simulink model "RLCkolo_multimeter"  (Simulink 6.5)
settings: Solver=ode45  StartTime=0.0  StopTime=1  RelTol=1e-6
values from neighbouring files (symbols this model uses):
  A = [-R/L -1/L; 1/C 0]    [primer_7_4c.m]
  C = str2num(C)    [patuvacki_bran_1.m]    (also in primer_7_3.m = 0.0001; primer_7_4.m = 0.0001; primer_7_4a.m = 0.0001; primer_7_4c.m = 0.0001)
undefined symbols (not defined in the file or in its folder): B, blocks, Continuous, D, powergui, x0, ZData
libraries: powerlib x8

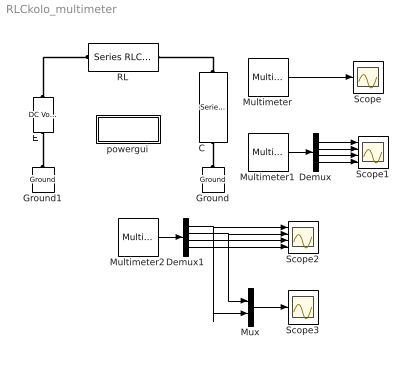
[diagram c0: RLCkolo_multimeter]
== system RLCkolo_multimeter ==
  C : powerlib/Elements/Series RLC Branch  Orientation=down  DialogController=PMDialogs.PMDefaultMaskDlg  PhysicalDomain=powersysdomain  SubClassName=unknown  LeftPortType=p1  RightPortType=p1  LConnTagsString=__new0  RConnTagsString=__new0  BranchType=C  Resistance=1  Inductance=1e-3  SetiL0=off  InitialCurrent=0  Capacitance=100e-6  Setx0=on  InitialVoltage=0  Measurements=Branch voltage and current
  Demux : Demux
  Demux1 : Demux
  E : powerlib/Electrical Sources/DC Voltage Source  Orientation=up  DialogController=PMDialogs.PMDefaultMaskDlg  SystemSampleTime=-1  Amplitude=12  Measurements=None
  Ground : powerlib/Elements/Ground  Orientation=down  DialogController=PMDialogs.PMDefaultMaskDlg  PhysicalDomain=powersysdomain  SubClassName=unknown  LeftPortType=p1  RightPortType=p1  LConnTagsString=a
  Ground1 : powerlib/Elements/Ground  Orientation=down  DialogController=PMDialogs.PMDefaultMaskDlg  PhysicalDomain=powersysdomain  SubClassName=unknown  LeftPortType=p1  RightPortType=p1  LConnTagsString=a
  Multimeter : powerlib/Measurements/Multimeter  SystemSampleTime=-1  PhasorSimulation=off  OutputType=Complex  sel=[1 2 3 4]  L=4  Gain=[1 1 1 1]  yselected={'Ub: C','Ub: RL','Ib: C','Ib: RL'};  PSBOutputType=1  PSBequivalent=0  AxesSetting=[0,0.1,-100,100]  Display=0  SavedBlockNames=-11
  Multimeter1 : powerlib/Measurements/Multimeter  SystemSampleTime=-1  PhasorSimulation=off  OutputType=Complex  sel=[1 2 3 4]  L=4  Gain=[1 1 1 1]  yselected={'Ub: C','Ub: RL','Ib: C','Ib: RL'};  PSBOutputType=1  PSBequivalent=0  AxesSetting=[0,0.1,-100,100]  Display=0  SavedBlockNames=-11
  Multimeter2 : powerlib/Measurements/Multimeter  SystemSampleTime=-1  PhasorSimulation=off  OutputType=Complex  sel=[1 2 3 4]  L=4  Gain=[1 1 1 1]  yselected={'Ub: C','Ub: RL','Ib: C','Ib: RL'};  PSBOutputType=1  PSBequivalent=0  AxesSetting=[0,0.1,-100,100]  Display=0  SavedBlockNames=-11
  Mux : Mux  Inputs=2
  RL : powerlib/Elements/Series RLC Branch  DialogController=PMDialogs.PMDefaultMaskDlg  PhysicalDomain=powersysdomain  SubClassName=unknown  LeftPortType=p1  RightPortType=p1  LConnTagsString=__new0  RConnTagsString=__new0  BranchType=RL  Resistance=3.6  Inductance=0.57  SetiL0=on  InitialCurrent=0  Capacitance=100e-6  Setx0=on  InitialVoltage=0  Measurements=Branch voltage and current
  Scope : Scope
  Scope1 : Scope  NumInputPorts=4
  Scope2 : Scope  NumInputPorts=4
  Scope3 : Scope
  powergui : Subsystem  AncestorBlock=powerlib/powergui  InitFcn=powergui( 'InitFcn_Callback' , gcb , 0 , [ ] );  mask(PSB option menu block){SimulationMode=Continuous, SampleTime=50e-6, echomessages=off, RestoreLinks=warning, x0status=blocks, Frange=[0:2:500], Ylog=off, Xlog=on, ShowGrid=off, save=off, variable=ZData, structure=, ZoomFFT=on, StartTime=0.0, cycles=1, DisplayStyle=1, fundamental=60, FreqAxis=off, MaxFrequency=1000, frequencyindice=0, frequencyindicesteady=1, RmsSteady=1, display=off, Ts=0, frequency=60, methode=off, HookPort=off, Interpol=off}
      mask prompts: SimulationMode "Simulation mode"; SampleTime "Sample time Ts (when simulation mode is Discrete) (s)"; echomessages "Echo  Messages"; RestoreLinks "Restore disabled links"; x0status "Initial electrical states status"; Frange "Impedance tool: Frequency Range"; Ylog "Impedance tool: Log impedance"; Xlog "Impedance tool: log Frequency"; ShowGrid "Impedance tool: grid"; save "Impedance tool: Save Data To Workspace"; variable "Impedance tool: Variable Name"; structure "Structure Name (PSBFFTSCOPE)"; ZoomFFT "ZoomFFT (PSBFFTSCOPE)"; StartTime "Start Time (PSBFFTSCOPE)"; cycles "Cycles (PSBFFTSCOPE)"; DisplayStyle "Display style (PSBFFTSCOPE)"; fundamental "Fundamental (PSBFFTSCOPE)"; FreqAxis "Frequency Axis (PSBFFTSCOPE)"; MaxFrequency "Max Frequency (PSBFFTSCOPE)"; frequencyindice "Load flow frequency (Hz)"; frequencyindicesteady "Frequency indice (STEADYSTATE)"; RmsSteady "RMS display (STEADYSTATE)"; display "Display Results"; Ts "OBSOLETE 1"; frequency "Phasor frequency (Hz)"; methode "Phasor simulation"; HookPort "Hook port"; Interpol "Interpolate"
      mask init:
      | powerlibroot = which('powersysdomain');
      | PSBroot = powerlibroot(1:end-16);
      | %
      | switch SimulationMode
      | 	case 1
      | 		message=sprintf('Continuous');
      | 	case 2
      |         SampleTimeeval=evalin('base',SampleTime,'NaN');
      |         if isnan(SampleTimeeval)
      |             message=sprintf('Warning !!,\nUndefined sample time');
      |         else
      |             message=sprintf('Discrete,\nTs = %.4g s.',SampleTimeeval);
      |         end
      | 	case 3
      | 		message=sprintf('Phasors');
      | end
      | if strcmp(bdroot,'powerlib')
      |   message='powergui';
      | end
      | power_initmask();
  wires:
  Multimeter/1 -> Scope/1
  Multimeter1/1 -> Demux/1
  Demux/1 -> Scope1/1
  Demux/2 -> Scope1/2
  Demux/3 -> Scope1/3
  Demux/4 -> Scope1/4
  Multimeter2/1 -> Demux1/1
  Demux1/1 -> Scope2/1, Mux/2
  Demux1/2 -> Scope2/2, Mux/1
  Demux1/3 -> Scope2/3
  Demux1/4 -> Scope2/4
  Mux/1 -> Scope3/1
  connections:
  C/LConn1 -- RL/RConn1
  E/RConn1 -- RL/LConn1
  Ground/LConn1 -- C/RConn1
  Ground1/LConn1 -- E/LConn1

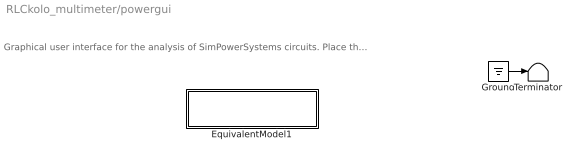
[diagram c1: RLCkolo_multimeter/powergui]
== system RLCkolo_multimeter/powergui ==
  note: Graphical user interface for the analysis of SimPowerSystems circuits. Place the Powergui block in the top-level of your model and double-click on it to open the GUI.
  EquivalentModel1 : Subsystem
  Ground : Ground
  Terminator : Terminator
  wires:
  Ground/1 -> Terminator/1

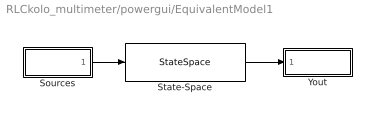
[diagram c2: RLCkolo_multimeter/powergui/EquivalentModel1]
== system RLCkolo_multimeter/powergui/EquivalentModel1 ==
  Sources : Subsystem
  State-Space : StateSpace  A=A  B=B  C=C  D=D  X0=x0
  Yout : Subsystem
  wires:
  Sources/1(u) -> State-Space/1
  State-Space/1 -> Yout/1(v,i)

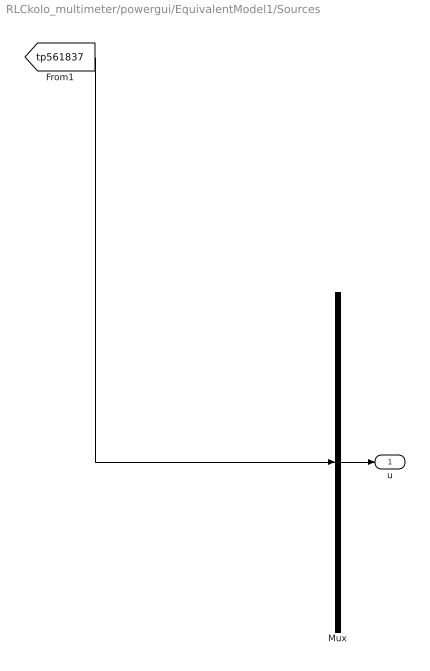
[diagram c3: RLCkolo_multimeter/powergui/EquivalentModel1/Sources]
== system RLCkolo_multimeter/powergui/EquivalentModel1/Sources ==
  Mux : Mux  Inputs=1
  u : Outport
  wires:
  Mux/1 -> u/1
  [tp561837] -> Mux/1

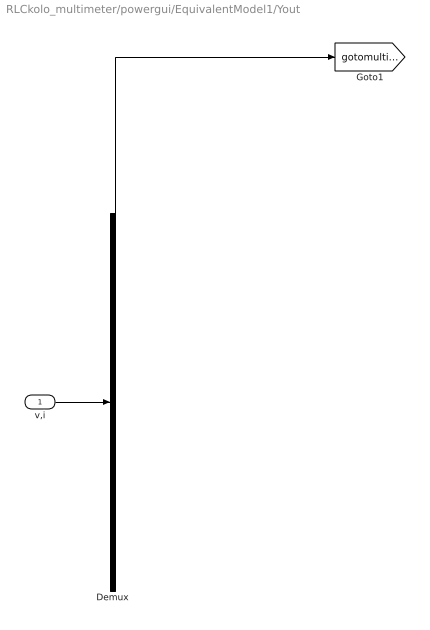
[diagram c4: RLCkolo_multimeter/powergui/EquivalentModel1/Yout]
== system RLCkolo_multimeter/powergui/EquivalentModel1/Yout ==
  v,i : Inport
  Demux : Demux  Outputs=1
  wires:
  v,i/1 -> Demux/1
  Demux/1 -> [gotomultimeterPSB]
